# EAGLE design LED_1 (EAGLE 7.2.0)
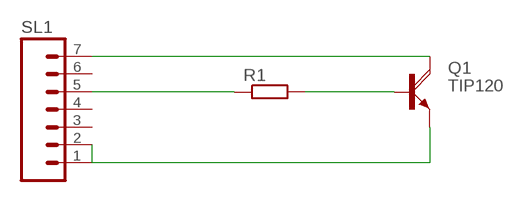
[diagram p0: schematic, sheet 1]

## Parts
Q1  TIP120  [TO220AH]
R1  R-EU_0204/7  [0204/7]
SL1  M07  [07P]

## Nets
N$1: Q1.B R1.2
N$2: Q1.C SL1.7
N$3: Q1.E SL1.1 SL1.2
N$4: R1.1 SL1.5
Unconnected: SL1.3 SL1.4 SL1.6

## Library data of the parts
Q1 = transistor-power:TIP120: NPN DARLINGTON TRANSISTOR
R1 = rcl:R-EU_: RESISTOR, European symbol
SL1 = con-amp-quick:M07: AMP QUICK CONNECTOR; OC_FARNELL: unknown; OC_NEWARK: unknown

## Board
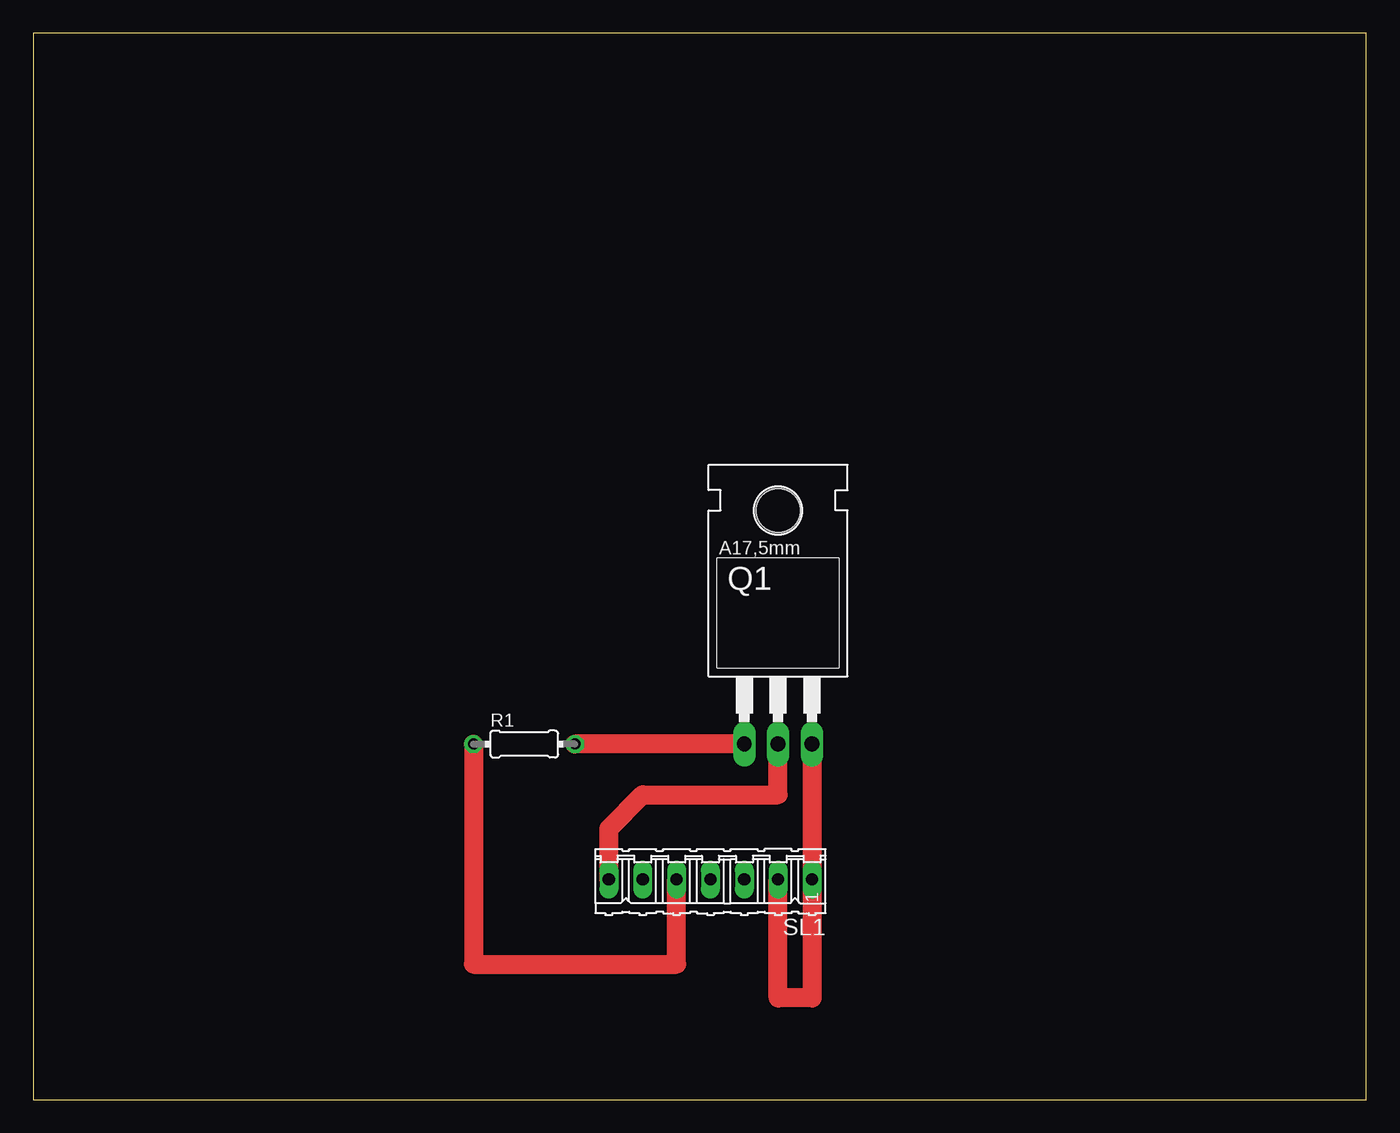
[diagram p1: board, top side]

Size 100 x 80 mm. Coordinates in mm from the lower left corner, seen from the top.
Outline: 0,0 100,0 100,80 0,80 0,0
Copper layers (1*16): Top 0.035mm / dielectric 1.5mm / Bottom 0.035mm
Design rules "default": minimum track width 10mil, minimum drill 24mil, track to track 8mil, track to pad 8mil, pad to pad 8mil, via to via 8mil, smd to smd 8mil, copper to edge 40mil, drill to drill 8mil, minimum pad ring 10mil, minimum via ring 8mil, stop-mask expansion 4mil, vias tented up to drill 0mil, thermal gap 10mil

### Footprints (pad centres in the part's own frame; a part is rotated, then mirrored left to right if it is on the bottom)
TO220AH = drill 1.118 long: B -2.54,-6.35; C 0,-6.35; E 2.54,-6.35 | hole 3.302: 0,11.176
0204/7 = drill 0.813 octagon: 1 -3.81,0; 2 3.81,0
07P = drill 0.914 long: 1 -7.62,0; 2 -5.08,0; 3 -2.54,0; 4 0,0; 5 2.54,0; 6 5.08,0; 7 7.62,0

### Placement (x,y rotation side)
Q1  55.88,33.02 0 top
R1  36.83,26.67 0 top
SL1  50.8,16.51 180 top

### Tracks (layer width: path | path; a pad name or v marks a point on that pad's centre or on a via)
N$1
  Top 1.422: Q1.B R1.2
N$2
  Top 1.422: SL1.7 43.18,20.32 45.72,22.86 55.88,22.86 Q1.C
N$3
  Top 1.422: Q1.E SL1.1 58.42,7.62 55.88,7.62 SL1.2
N$4
  Top 1.422: R1.1 33.02,10.16 48.26,10.16 SL1.5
